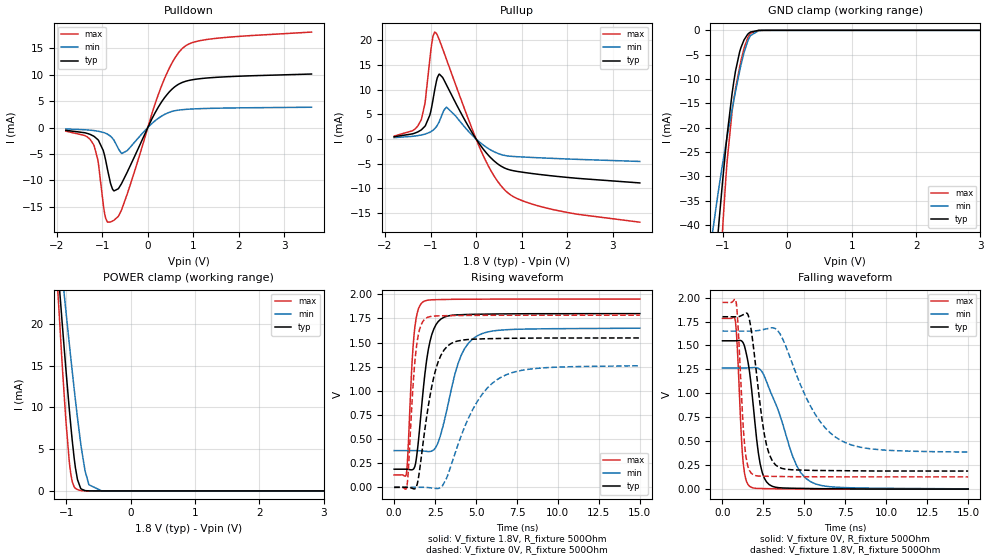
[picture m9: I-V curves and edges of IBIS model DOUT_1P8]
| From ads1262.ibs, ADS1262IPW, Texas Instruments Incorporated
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|   Model DOUT_1P8
[Model]   DOUT_1P8
Model_type   3-state
Polarity   Non-Inverting
Enable   Active-Low
Vmeas = 0.9
Vref = 1.8
Cref = 15pF
Rref = 500
|   typ   min   max
|   (slow PVT)   (nom PVT)   (fast PVT)
C_comp   0.308p   0.264p   0.323p
|C_comp (ON state)   0.308p   0.269p   0.326p
|C_comp (OFF state)   0.308p   0.264p   0.323p
| Where   nom PVT is  Nominal Process, 1.8V, 27C
|   Fast PVT is Strong Process, 1.65V, -40C
|   Slow PVT is Weak Process, 1.95V, 125C
[Voltage Range]   1.8   1.65   1.95
[Temperature Range]   27   125   -40
[Pullup Reference]   1.8   1.65   1.95
[Pulldown Reference]   -0   -0   -0
[Power Clamp Reference]   1.8   1.65   1.95
[GND Clamp Reference]   -0   -0   -0
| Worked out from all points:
|   slope of the pulldown table from 0 to 0.27 V, typ, clamps not added: 61.2 ohm
|   slope of the pullup table from 0 to 0.27 V, typ, clamps not added: 82.1 ohm
|   GND clamp passes 1 mA (typ) near -0.63 V on its own axis
|   POWER clamp passes 1 mA (typ) near -0.81 V on its own axis
|   falling waveform, V_fixture 0V, R_fixture 500Ohm: 20-80 % time 616ps typ, 1.56ns min, 304ps max; typ from 1.55 V to 0.001 V
|   rising waveform, V_fixture 1.8V, R_fixture 500Ohm: 20-80 % time 647ps typ, 1.19ns min, 341ps max; typ from 0.188 V to 1.8 V
|   rising waveform, V_fixture 0V, R_fixture 500Ohm: 20-80 % time 914ps typ, 2.06ns min, 414ps max; typ from 0 V to 1.55 V
|   falling waveform, V_fixture 1.8V, R_fixture 500Ohm: 20-80 % time 733ps typ, 2.2ns min, 348ps max; typ from 1.8 V to 0.189 V
[Pulldown]
|   Voltage   I(typ)   I(min)   I(max)
-1.8V     -529.4uA   -266.9uA   -685.6uA
-1.384V   -985.4uA   -419.1uA   -1.504mA
-1.184V   -1.647mA   -575.5uA   -3.318mA
-1.093V   -2.335mA   -692.9uA   -6.355mA
-941.4mV  -5.56mA    -1.032mA   -16.57mA
-817.2mV  -10.63mA   -1.652mA   -17.9mA
-741.6mV  -12.02mA   -2.417mA   -17.57mA
-568.8mV  -10.5mA    -4.928mA   -15.46mA
252mV     4.169mA    1.878mA    6.748mA
759.6mV   8.559mA    3.387mA    15.01mA
1.364V    9.436mA    3.634mA    16.77mA
3.595V    10.14mA    3.847mA    18.1mA
[GND Clamp]
|   Voltage   I(typ)   I(min)   I(max)
-1.8V     -173.9mA   -111.9mA   -255.2mA
-1.222V   -65.42mA   -47.17mA   -94.62mA
-1.098V   -44.82mA   -35.32mA   -62.42mA
-1.066V   -39.75mA   -32.42mA   -54.43mA
-1.006V   -30.89mA   -27.35mA   -40.61mA
-936mV    -21.42mA   -21.86mA   -26.78mA
-860.4mV  -13.06mA   -16.34mA   -16.76mA
-833.4mV  -10.56mA   -14.43mA   -14.2mA
-720mV    -3.482mA   -7.033mA   -6.176mA
-574.2mV  -351.6uA   -1.081mA   -624.8uA
-358.2mV  -1.049uA   -10.75uA   -582.5nA
3.595V    0A         0A         0A
[Pullup]
|   Voltage   I(typ)   I(min)   I(max)
-1.8V     460.9uA    288.7uA    598.5uA
-1.395V   1.052mA    551.6uA    1.685mA
-1.206V   1.842mA    809.4uA    3.883mA
-1.12V    2.644mA    1.003mA    7.476mA
-1.017V   4.828mA    1.366mA    16.07mA
-909mV    9.955mA    2.095mA    21.63mA
-806.4mV  13.13mA    3.591mA    20.01mA
-649.8mV  10.93mA    6.453mA    16.08mA
154.8mV   -2.018mA   -1.194mA   -3.319mA
646.2mV   -5.95mA    -3.349mA   -10.46mA
1.591V    -7.374mA   -3.877mA   -14.06mA
3.595V    -8.877mA   -4.533mA   -16.82mA
[POWER Clamp]
|   Voltage   I(typ)   I(min)   I(max)
-1.8V     87.39mA    77.2mA     101.7mA
-1.363V   49.57mA    48.23mA    53.69mA
-1.066V   20.13mA    25.93mA    15.19mA
-1.017V   15.45mA    22.26mA    9.469mA
-946.8mV  9.094mA    17.05mA    2.939mA
-909mV    6.034mA    14.32mA    1.106mA
-828mV    1.363mA    8.776mA    156.6uA
-779.4mV  329.8uA    5.798mA    51.92uA
-709.2mV  34.25uA    2.374mA    8.078uA
-649.8mV  5.575uA    736.1uA    1.353uA
-450mV    0A         3.178uA    0A
3.595V    0A         0A         0A
[Ramp]
R_load = 500
|   typ   min   max
dV/dt_r   0.966883/6.4689e-10   0.760567/1.192e-09   1.09301/3.41386e-10
dV/dt_f   0.928469/6.1613e-10   0.756817/1.56255e-09   1.06962/3.0387e-10
[Falling Waveform]
V_fixture = 0V
V_fixture_min = 0V
V_fixture_max = 0V
R_fixture = 500Ohm
C_fixture = 0F
|   Time   V(typ)   V(min)   V(max)
0s        1.549V     1.265V     1.783V
789.3ps   1.549V     1.265V     1.758V
1.212ns   1.54V      1.265V     383mV
1.413ns   1.447V     1.265V     111.6mV
1.641ns   1.237V     1.267V     32.14mV
2.301ns   263.2mV    1.249V     6.858mV
3.047ns   29.4mV     970.6mV    4.366mV
4.539ns   8.805mV    241.5mV    2.068mV
5.384ns   6.645mV    77.37mV    1.308mV
15ns      1.236mV    3.187mV    39.83uV
[Rising Waveform]
V_fixture = 1.8V
V_fixture_min = 1.65V
V_fixture_max = 1.95V
R_fixture = 500Ohm
C_fixture = 0F
|   Time   V(typ)   V(min)   V(max)
0s        187.7mV    380.5mV    128.3mV
743.1ps   187.7mV    380.4mV    138mV
1.212ns   196.5mV    380.4mV    1.573V
1.413ns   373.4mV    380.4mV    1.808V
1.746ns   958.6mV    377mV      1.919V
2.086ns   1.427V     370.3mV    1.939V
2.561ns   1.687V     421.1mV    1.944V
3.906ns   1.787V     1.284V     1.948V
5.084ns   1.793V     1.57V      1.949V
15ns      1.799V     1.648V     1.95V
[Rising Waveform]
V_fixture = 0V
V_fixture_min = 0V
V_fixture_max = 0V
R_fixture = 500Ohm
C_fixture = 0F
|   Time   V(typ)   V(min)   V(max)
0s        1.029nV    3.208nV    730.2pV
766.2ps   187.4uV    112.5uV    842.8uV
1.153ns   -13.25mV   169.3uV    1.05V
1.342ns   -588.3uV   197uV      1.429V
1.877ns   601.4mV    219.8uV    1.743V
2.691ns   1.302V     -11.22mV   1.776V
3.639ns   1.503V     309.8mV    1.78V
5.084ns   1.536V     891.2mV    1.781V
6.584ns   1.542V     1.145V     1.782V
15ns      1.547V     1.259V     1.783V
[Falling Waveform]
|Gnd
V_fixture = 1.8V
V_fixture_min = 1.65V
V_fixture_max = 1.95V
R_fixture = 500Ohm
C_fixture = 0F
|   Time   V(typ)   V(min)   V(max)
0s        1.8V       1.65V      1.95V
819.8ps   1.799V     1.65V      1.965V
1.342ns   1.828V     1.65V      478mV
1.614ns   1.791V     1.65V      209.9mV
1.877ns   1.505V     1.65V      150.5mV
2.691ns   458.8mV    1.673V     134.7mV
3.439ns   229.2mV    1.639V     132.4mV
5.384ns   196.4mV    862.8mV    129.7mV
7.184ns   193mV      512.6mV    128.6mV
15ns      189.2mV    387.3mV    128.3mV
